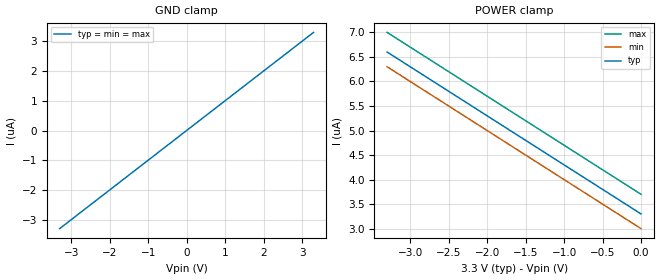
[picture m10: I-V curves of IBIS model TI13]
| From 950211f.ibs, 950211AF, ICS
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|   Model TI13
[Model]   TI13
Model_type   Input
Polarity   Inverting
Vinl = 800.00mV
Vinh =   2.00V
C_comp   5.50pF   5.00pF   6.00pF
[Temperature Range]   27.00   70.00   0.00
[Voltage Range]   3.30V   3.00V   3.70V
[GND_clamp]
| voltage   I(typ)   I(min)   I(max)
-3.3V     -3.3uA     -3.3uA     -3.3uA
1.3V      1.3uA      1.3uA      1.3uA
1.6V      1.6uA      1.6uA      1.6uA
3.3V      3.3uA      3.3uA      3.3uA
[POWER_clamp]
| voltage   I(typ)   I(min)   I(max)
-3.3V     6.6uA      6.3uA      7uA
-3.1V     6.4uA      6.1uA      6.8uA
-1.9V     5.2uA      4.9uA      5.6uA
0V        3.3uA      3uA        3.7uA
